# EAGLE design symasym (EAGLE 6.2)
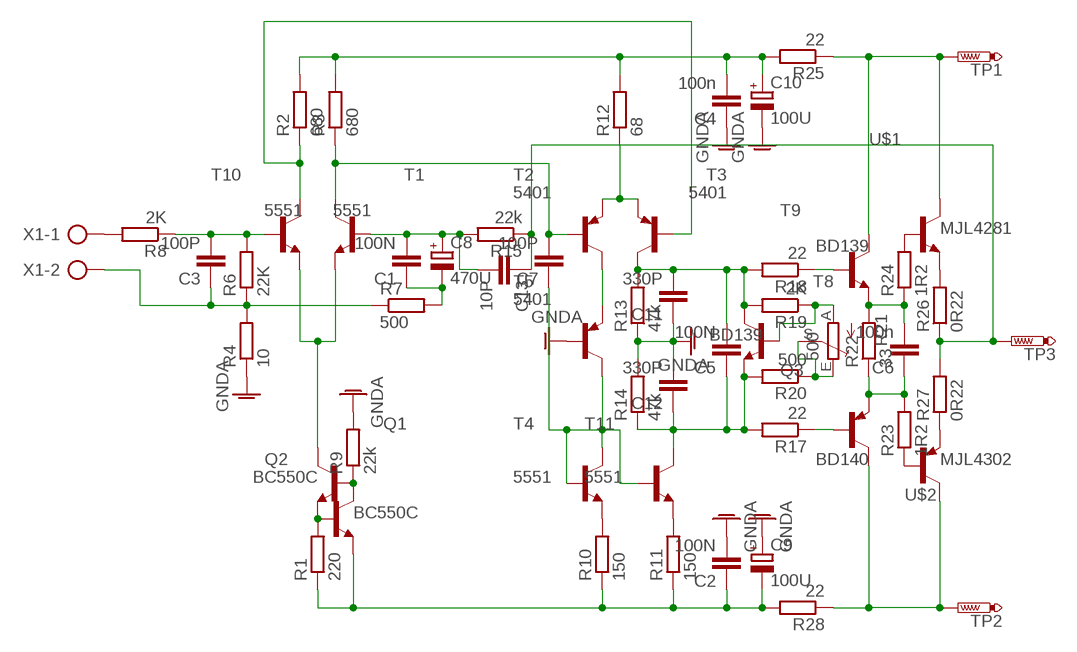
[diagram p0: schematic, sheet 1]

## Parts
C1  100N  C5/2.5  [C5B2.5]
C2  100N  C5/2.5  [C5B2.5]
C3  100P  C5/2.5  [C5B2.5]
C4  100n  C5/2.5  [C5B2.5]
C5  100N  C5/2.5  [C5B2.5]
C6  100n  C5/2.5  [C5B2.5]
C7  100P  C5/2.5  [C5B2.5]
C8  470U  CPOL-EUE5-13  [E5-13]
C9  100U  CPOL-EUE5-13  [E5-13]
C10  100U  CPOL-EUE5-13  [E5-13]
C11  330P  C5/2.5  [C5B2.5]
C12  330P  C5/2.5  [C5B2.5]
C13  10P  C5/2.5  [C5B2.5]
Q1  BC550C  [TO92-EBC]
Q2  BC550C  [TO92-EBC]
Q3  BD140  [TO126]
R1  220  R-EU_0207/12  [0207/12]
R2  680  R-EU_0207/12  [0207/12]
R3  680  R-EU_0207/12  [0207/12]
R4  10  R-EU_0207/12  [0207/12]
R6  22K  R-EU_0207/12  [0207/12]
R7  500  R-EU_0207/12  [0207/12]
R8  2K  R-EU_0207/12  [0207/12]
R9  22k  R-EU_0207/12  [0207/12]
R10  150  R-EU_0207/12  [0207/12]
R11  150  R-EU_0207/12  [0207/12]
R12  68  R-EU_0207/12  [0207/12]
R13  47k  R-EU_0207/12  [0207/12]
R14  47k  R-EU_0207/12  [0207/12]
R15  22k  R-EU_0207/10  [0207/10]
R17  22  R-EU_0207/12  [0207/12]
R18  22  R-EU_0207/10  [0207/10]
R19  2K  R-EU_0207/12  [0207/12]
R20  500  R-EU_0207/12  [0207/12]
R21  500  TRIM_EU-B64Y  [B64Y]
R22  33  R-EU_0411/15  [0411/15]
R23  1R2  R-EU_0411/15  [0411/15]
R24  1R2  R-EU_0411/15  [0411/15]
R25  22  R-EU_0411/15  [0411/15]
R26  0R22  R-EU_0922/22  [0922/22]
R27  0R22  R-EU_0922/22  [0922/22]
R28  22  R-EU_0411/15  [0411/15]
T1  5551  2N5551-NPN-TO92-EBC  [TO92-EBC]
T2  5401  2N5401-PNP-TO92-EBC  [TO92-EBC]
T3  5401  2N5401-PNP-TO92-EBC  [TO92-EBC]
T4  5551  2N5551-NPN-TO92-EBC  [TO92-EBC]
T5  5401  2N5401-PNP-TO92-EBC  [TO92-EBC]
T8  BD139  [TO126]
T9  BD139  [TO126]
T10  5551  2N5551-NPN-TO92-EBC  [TO92-EBC]
T11  5551  2N5551-NPN-TO92-EBC  [TO92-EBC]
TP1  PTR1PAD1-17Y  [P1-17Y]
TP2  PTR1PAD1-17Y  [P1-17Y]
TP3  PTR1PAD1-17Y  [P1-17Y]
U$1  MJL4281  [TO-264]
U$2  MJL4302  [TO-264]
X1  AK500/2  [AK500/2]

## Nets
GNDA: C2.2 C4.1 C9.+ C10.- C11.1 C12.2 R4.1 R9.2 R13.1 R14.2 T5.B
N$1: Q1.E Q2.B R1.2
N$2: Q1.B Q2.C R9.1
N$3: R2.1 T3.B T10.C
N$4: C3.1 R4.2 R6.1 R7.1 X1.2
N$5: C7.2 R3.1 T1.C T2.B
N$6: R10.2 T4.E
N$7: Q1.C T1.E T10.E
N$8: C4.2 C10.+ R2.2 R3.2 R12.2 R25.2
N$9: C3.2 R6.2 R8.1 T10.B
N$10: C7.1 T4.B T4.C T5.C T11.B
N$11: R11.2 T11.E
N$13: T2.C T5.E
N$14: R12.1 T2.E T3.E
N$15: C2.1 C9.- Q2.E R1.1 R10.1 R11.1 R28.2
N$16: C1.1 C8.- R7.2
N$17: C1.2 C8.+ C13.2 R15.2 T1.B
N$18: C5.1 C12.1 R14.1 R17.2 R20.2 T8.1(E) T11.C
N$19: C13.1 R15.1 R26.1 R27.2 TP3.TP
N$20: C5.2 C11.2 R13.2 R18.2 R19.2 T3.C T8.2(C)
N$21: R25.1 T9.2(C) TP1.TP U$1.C
N$23: R8.2 X1.1
N$24: Q3.2(C) R28.1 TP2.TP U$2.C
N$26: R19.1 R21.A T8.3(B)
N$27: R20.1 R21.E R21.S
N$28: R18.1 T9.3(B)
N$29: Q3.3(B) R17.1
N$30: C6.1 Q3.1(E) R22.1 R23.2
N$31: C6.2 R22.2 R24.1 T9.1(E)
N$32: R24.2 U$1.B
N$33: R23.1 U$2.B
N$34: R26.2 U$1.E
N$36: R27.1 U$2.E

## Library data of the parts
C1-C7 C11-C13 = capacitor-wima:C: CAPACITOR
C8-C10 = rcl:CPOL-EU: POLARIZED CAPACITOR, European symbol
Q1 Q2 = transistor-npn:BC550*: NPN Transistor
Q3 = transistor-pnp:BD140: PNP Transistor
R1-R4 R6-R15 R17-R20 R22-R28 = resistor:R-EU_: RESISTOR, European symbol
R21 = pot:TRIM_EU-: POTENTIOMETER
T1 T4 T10 T11 = transistor-neu-to92:*-NPN-: NPN Transistror
T2 T3 T5 = transistor-neu-to92:*-PNP-: PNP Transistror
T8 T9 = transistor:BD139: NPN TRANSISTOR
TP1-TP3 = testpad:PTR1: TEST PIN
U$1 = Rudi_TO264:MJL4281: MJL4281 NPN BCE TO-264
U$2 = Rudi_TO264:MJL4302: MJL4302 PNP BCE TO-264
X1 = con-ptr500:AK500/2: CONNECTOR; OC_FARNELL: unknown; OC_NEWARK: unknown

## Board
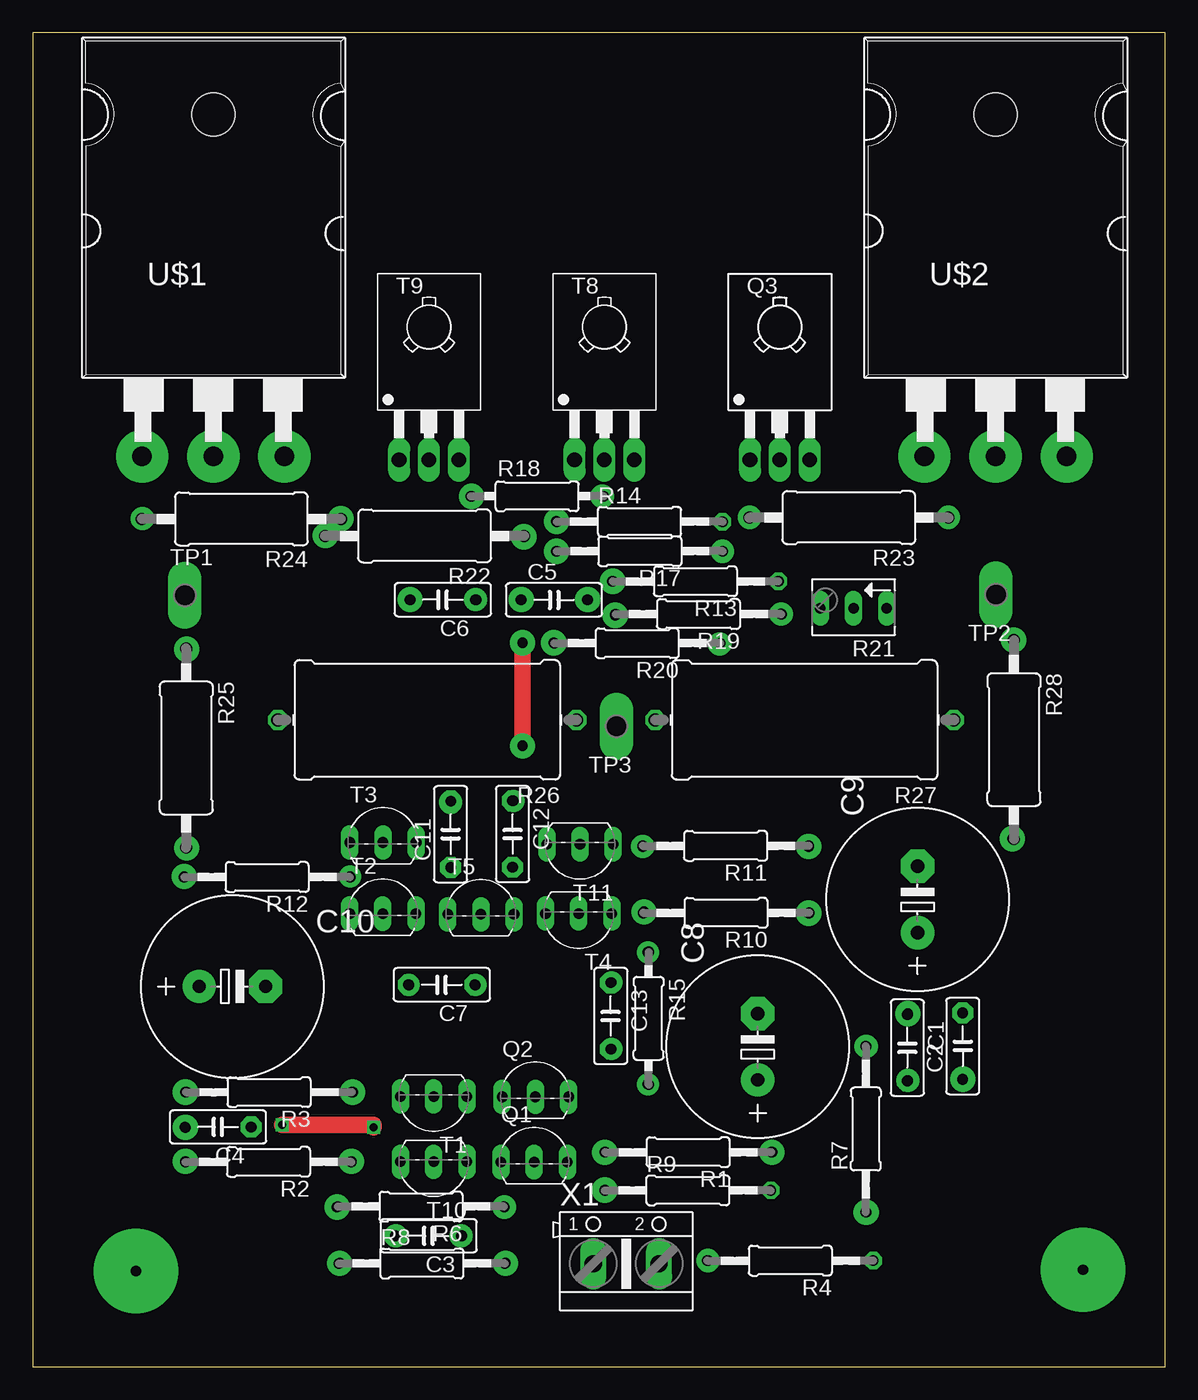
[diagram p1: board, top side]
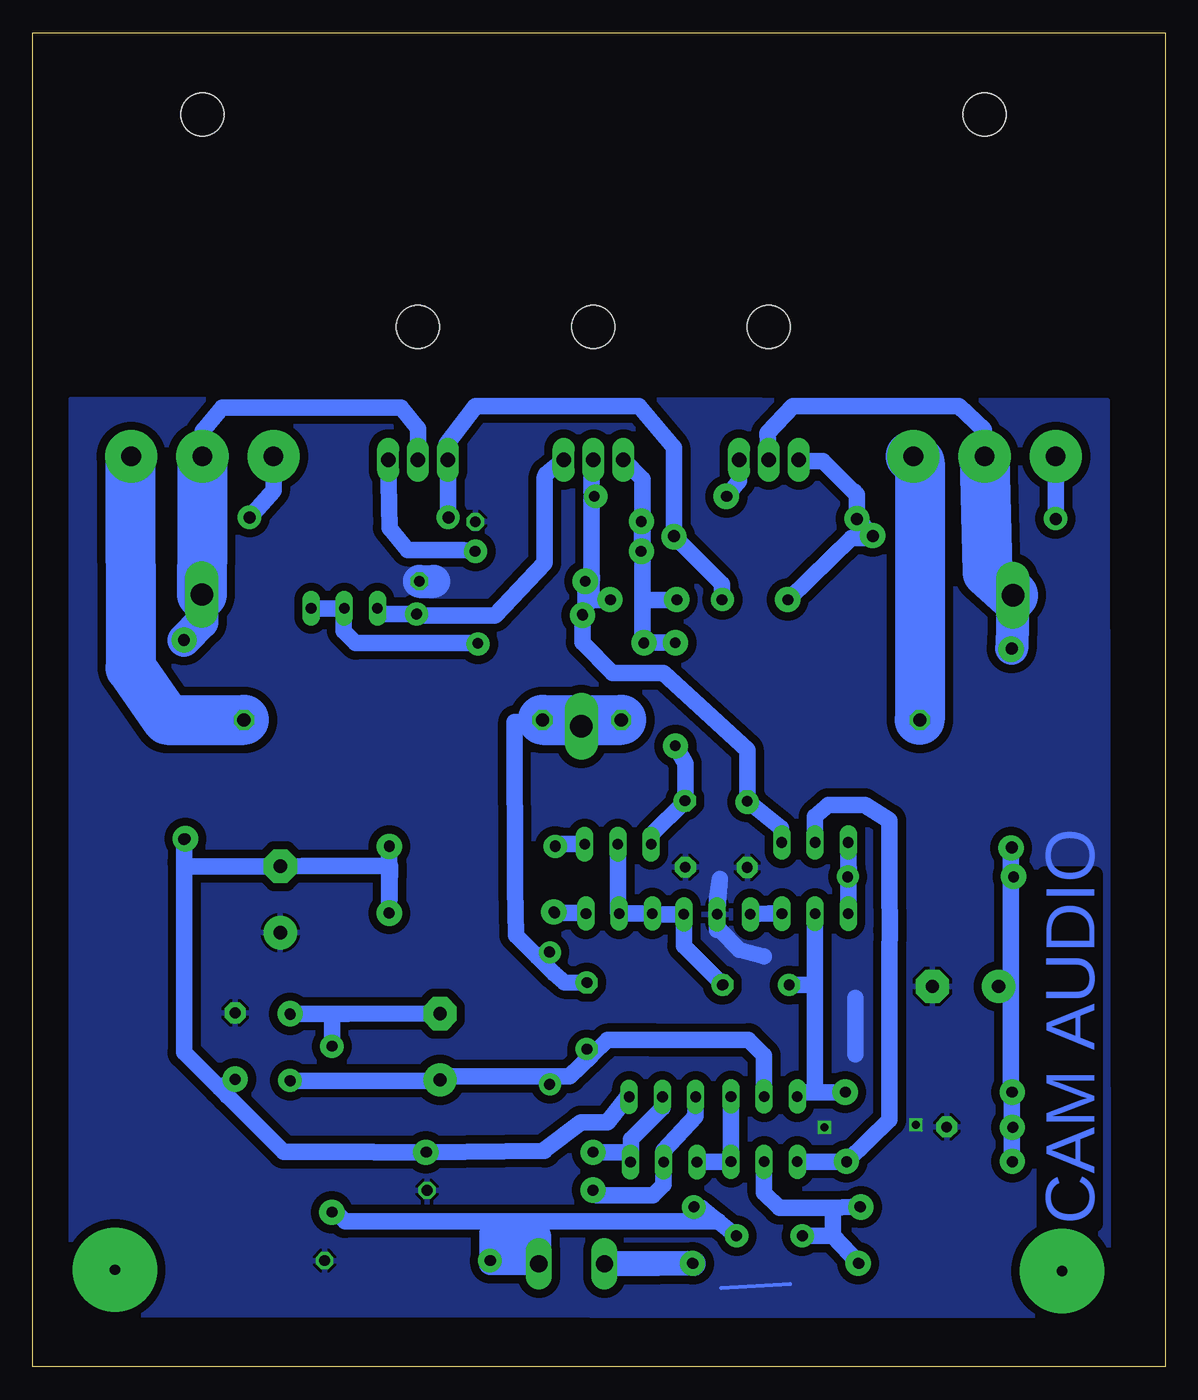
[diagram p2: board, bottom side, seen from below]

Size 86.7 x 102.13 mm. Coordinates in mm from the lower left corner, seen from the top.
Outline: 0,0 86.7,0 86.7,102.13 0,102.13 0,0
Copper layers (1*16): Top 0.035mm / dielectric 1.5mm / Bottom 0.035mm
Design rules: minimum track width 10mil, minimum drill 24mil, track to track 25mil, track to pad 25mil, pad to pad 25mil, via to via 25mil, smd to smd 25mil, copper to edge 40mil, drill to drill 8mil, minimum pad ring 10mil, minimum via ring 8mil, stop-mask expansion 4mil, vias tented up to drill 0mil, thermal gap 10mil

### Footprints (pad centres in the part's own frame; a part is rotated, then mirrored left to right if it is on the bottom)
C5B2.5 = drill 0.813 pad 1.6 octagon: 1 -2.54,0; 2 2.54,0
E5-13 = drill 1.016 pad 2.54: + -2.54,0 | drill 1.016 pad 2.54 octagon: - 2.54,0
TO92-EBC = drill 0.813 long: B 0,-1.27; C -2.54,-1.27; E 2.54,-1.27
TO126 = drill 1.118 long: 1 -2.286,-5.08; 2 0,-5.08; 3 2.286,-5.08 | hole 3.302: 0,5.08
0207/12 = drill 0.813 octagon: 1 -6.35,0; 2 6.35,0
0207/10 = drill 0.813 octagon: 1 -5.08,0; 2 5.08,0
B64Y = drill 0.813 long: A 2.54,0; E -2.54,0; S 0,0
0411/15 = drill 0.914 octagon: 1 -7.62,0; 2 7.62,0
0922/22 = drill 1.016 octagon: 1 -11.43,0; 2 11.43,0
TO92-EBC' = drill 0.813 long: B 0,-1.27; C 2.54,-1.27; E -2.54,-1.27
P1-17Y = drill 1.702 pad 2.121 long: TP 0,0
TO-264 = drill 1.5 pad 4: B -5.45,-6.096; E 5.45,-6.096 | drill 1.499 pad 4: C 0,-6.096 | hole 3.3: 0,20.09
AK500/2 = drill 1.321 long: 1 -2.515,0; 2 2.515,0

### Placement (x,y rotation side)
C1  66.96,24.43 270 top
C2  71.2,24.55 90 top
C3  30.31,10.03 180 top
C4  14.19,18.36 180 top
C5  39.91,58.71 0 top
C6  31.4,58.72 180 top
C7  31.32,29.25 180 top
C8  55.51,24.5 90 top
C9  67.74,35.78 90 top
C10  15.29,29.12 0 top
C11  32,40.77 90 top
C12  36.74,40.79 270 top
C13  44.25,26.86 270 top
Q1  38.39,16.94 0 top
Q2  38.49,21.94 0 top
Q3  57.2,74.52 0 top
R1  50.18,16.43 180 top
R2  18.05,15.69 180 top
R3  18.1,21.03 180 top
R4  58,8.13 180 top
R6  29.72,12.27 180 top
R7  63.78,18.2 90 top
R8  29.8,7.91 0 top
R9  50.16,13.51 0 top
R10  53.08,34.75 180 top
R11  53.05,39.88 180 top
R12  17.95,37.49 180 top
R13  50.74,60.13 180 top
R14  46.46,64.69 0 top
R15  47.15,26.68 270 top
R17  46.48,62.43 180 top
R18  38.62,66.64 0 top
R19  50.97,57.62 180 top
R20  46.28,55.39 180 top
R21  62.84,58.06 180 top
R22  30,63.6 180 top
R23  62.48,65 180 top
R24  15.98,64.9 180 top
R25  11.75,47.37 270 top
R26  30.21,49.52 180 top
R27  59.09,49.52 180 top
R28  75.12,48.01 270 top
T1  5551  [TO92-EBC']  30.7,19.43 180 top
T2  5401  [TO92-EBC']  26.8,35.96 0 top
T3  5401  [TO92-EBC']  26.81,41.41 0 top
T4  5551  [TO92-EBC']  41.8,33.43 180 top
T5  5401  [TO92-EBC']  34.31,35.91 0 top
T8  43.77,74.52 0 top
T9  30.34,74.52 0 top
T10  5551  [TO92-EBC']  30.7,14.43 180 top
T11  5551  [TO92-EBC']  41.9,38.73 180 top
TP1  11.65,59.07 0 top
TP2  73.75,59.12 180 top
TP3  44.7,49.03 180 top
U$1  13.83,75.79 0 top
U$2  73.71,75.79 0 top
X1  45.44,7.89 0 top

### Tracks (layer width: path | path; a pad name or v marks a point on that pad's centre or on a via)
GNDA  (via drill 0.6)
  Top 1.27: v19.1,18.53 26.1,18.53 v26.1,18.33
  Bottom 0.305: 28.7,6.33 34,6.03
  Bottom 1.27: 34.1,37.33 34.3,35.83 | 34.1,37.33 34.2,36.33 34.3,35.83 | 34.3,35.83 34.3,33.43 34.1,33.43 32.6,31.93 30.7,31.43 | 34.1,37.33 T5.B | 23.7,28.23 23.7,23.93
  Bottom 2.54: R13.1 56,60.13
  pour Bottom: 4.44,73.98 83.73,74.08 83.73,4 4.34,3.9
N$1
  Bottom 1.27: R1.2 40.89,16.43 Q1.E 40.9,15.7 40.9,17.43 38.49,19.84 Q2.B
N$2
  Bottom 1.27: Q2.C 35.95,19.18 38.39,16.54 Q1.B | Q1.B 38.41,15.47 | Q1.B 38.41,15.45 38.41,13.92 39.2,13.13 43.53,13.13 R9.1
N$3
  Bottom 1.27: T3.B 26.8,42.13 25.8,43.03 23,43.03 21.1,41.83 21.1,36.65 21.09,33.44 21.1,31.73 21.1,18.89 R2.1 27.8,15.69 27.81,15.7 T10.C
N$4
  Bottom 1.016: 48.9,10.43 48.9,11.13
  Bottom 1.27: C3.1 35.49,12.17 R6.1 34.21,11.13 48.9,11.13 62.8,11.13 63.52,11.85 R7.1
  Bottom 1.778: X1.2 51.65,7.89 R4.2 51.6,8.13 51.6,10.43 50.6,10.43 50.6,9.13 50,9.13 50,10.13 47.9,10.13 47.9,8.03 48.9,8.03 48.9,10.43
N$5  (via drill 0.8 pad 1.93)
  Bottom 1.27: R3.1 v24.5,21.03 26.7,21.03 | 26.7,21.03 28.16,21.03 T1.C | T2.B 26.8,28.73 | 26.8,28.73 26.8,21.13 26.7,21.03 | 26.8,28.73 26.82,29.25 C7.2
N$6
  Bottom 1.27: R10.2 44.6,34.73 44.4,34.76 T4.E
N$7
  Bottom 1.27: 33.25,21.07 T1.E T10.E 35.82,15.7 Q1.C
N$8
  Bottom 1.27: 11.75,18.36 R3.2 11.8,21.08 11.8,29.73 | 11.75,18.36 11.75,15.74 R2.2 | 11.8,29.73 11.8,37.33 | 11.8,37.33 11.8,39.5 R25.2 | C10.+ 11.81,29.12 11.8,29.73 | R12.2 11.76,37.39 11.8,37.33 | C4.2 11.75,18.36
N$9
  Bottom 1.27: 25.45,12.17 R6.2 25.36,12.16 | 25.45,12.17 25.45,10.03 | 25.45,10.03 R8.1 | 25.45,12.17 29.54,12.17 30.7,13.33 T10.B | C3.2 25.45,10.03
N$10
  Bottom 1.27: 36.8,34.69 T5.C | T5.C 39.19,34.63 T4.C T4.B 41.9,34.8 T11.B | T5.C 36.85,32.24 C7.1
N$11
  Bottom 1.27: R11.2 46.65,39.88 46.3,40.03 44.4,40.04 T11.E
N$12  (via drill 0.8 pad 1.78)
  other vias: 36.1,12.23
N$13
  Bottom 1.27: T2.C 30.32,34.69 T5.E
N$14
  Bottom 1.27: T3.E 24.27,38.13 | 24.27,38.13 T2.E | R12.1 24.21,38.19 24.27,38.13
N$15
  Bottom 1.27: R1.1 60.53,16.43 | Q2.E 41.16,20.67 42.7,18.73 44.73,18.73 47.5,16.63 47.5,16.53 R1.1 | R11.1 59.43,39.85 R10.1 59.33,38.33 66.05,38.33 C9.- 74.81,38.32 75.12,38.63 | R1.1 60.65,16.45 67.5,16.45 71.78,20.73 | 71.8,20.73 71.78,20.73 | R28.2 75.12,38.63 | 75.12,38.63 75.12,24.07 72.39,21.34 | 72.39,21.34 71.78,20.73 | C2.1 72.39,21.34
N$16
  Bottom 0.813: 63.78,26.94 62.6,27.02
  Bottom 1.27: C8.- 62.6,27.02 66.87,27.02 C1.1 | R7.2 63.78,26.94
N$17
  Bottom 0.406: R15.2 45.6,22.2 45.6,22.23 | C13.2 43.93,24.32 43.93,23.84
  Bottom 1.27: T1.B 30.7,23.83 31.9,25.03 39.2,25.03 39.29,25.02 42.71,25.02 43.93,23.84 45.6,22.23 55.66,22.23 C8.+ 55.97,21.9 C1.2
N$18  (via drill 0.8 pad 1.93)
  Top 1.27: v37.5,55.43 v37.5,47.53
  Bottom 1.27: 40,55.32 40,58.63 | 40,58.63 40,61.73 | 40,61.73 40,62.03 | 40,62.03 40,67.96 T8.1 | R14.1 40.01,62.04 arc-90 40,62.03 | R17.2 40.03,61.7 arc90 40,61.73 | 37.25,58.59 C5.1 39.92,58.71 40,58.63 | 40,55.32 40,55.23 39.9,55.43 v37.5,55.43 | 40,55.32 R20.2 | v37.5,47.53 36.74,46.17 C12.1 39.36,40.71 T11.C
N$19
  Bottom 1.27: R26.1 49.8,49.38 49.78,36.63 49.7,33.03 48.1,31.43 | C13.1 45.98,29.43 46.8,30.13 48.1,31.43 | TP3.TP 46.75,49.43 R27.2 | R15.1 48.1,31.43
  Bottom 3.81: R27.2 R26.1
N$20  (via drill 0.6 pad 1.78)
  Bottom 1.27: 43.9,60.13 43.9,58.63 43.82,58.71 C5.2 | 43.9,60.13 43.9,60.53 | T8.2 43.9,69.31 43.9,66.97 | 43.9,66.97 v43.6,66.63 43.9,66.63 43.9,60.53 | 43.87,60.25 43.87,60.5 43.9,60.53 | 43.9,60.13 R13.2 44.39,58.15 R19.2 44.62,55.45 42.3,53.13 38.4,53.13 32,47.23 C11.2 29.41,41.24 T3.C | 43.9,66.97 R18.2
N$21
  Bottom 1.27: T9.2 30.44,71.49 28.5,73.53 15.8,73.53 13.9,71.73 13.9,69.76 U$1.C | TP1.TP 11.65,58.97
  Bottom 2.54: 11.65,58.97 R25.1
  Bottom 3.81: U$1.C 13.6,60.83 TP1.TP
N$22  (via drill 0.8 pad 1.78)
  other vias: 27.8,10.03
N$23
  Bottom 1.93: R8.2 38.87,7.89 X1.1
N$24  (via drill 0.8 pad 1.93)
  Bottom 1.27: 74.9,63.33 73.6,64.63 v73.8,59.13 74.9,68.5 U$2.C 73.7,69.7 73.7,71.63 72.2,73.43 58.5,73.43 57.2,71.83 Q3.2
  Bottom 2.54: TP2.TP 73.75,57 R28.1
  Bottom 3.81: U$2.C 73.71,63.74 TP2.TP
N$25  (via drill 0.8 pad 1.78)
  other vias: 33.9,58.73
N$26
  Bottom 1.27: T8.3 47.39,68.34 47.5,68.03 47.5,61.53 51.3,57.53 57.33,57.53 R19.1 60.16,57.62 R21.A
N$27
  Bottom 1.27: R21.E R21.S 62.9,57.9 62.9,56.33 61.96,55.39 R20.1
N$28
  Bottom 1.27: T9.3 32.63,67.8 R18.1
N$29
  Bottom 1.27: Q3.3 59.39,64.22 58,62.53 53.7,62.53 52.93,62.4 52.9,62.43 R17.1
N$30
  Bottom 1.27: R23.2 54.91,65.55 Q3.1 55,69.53 55,70.63 52.8,73.53 40.3,73.53 37.62,70.35 R22.1 33.94,59.92 C6.1
N$31
  Bottom 1.27: T9.1 27.91,69.44 27.8,69.33 26.2,69.33 23.7,66.83 23.73,66.89 | 23.73,66.89 23.8,67 | R24.1 23.5,64.8 22.5,63.46 24.02,63.46 C6.2 | R24.1 23.6,66.75 23.73,66.89 | R22.2 23.28,64.6 R24.1
N$32
  Bottom 1.27: U$1.B 8.38,64.92 R24.2
N$33
  Bottom 1.27: U$2.B 68.26,67.06 R23.1
N$34
  Bottom 1.27: R26.2 18.79,51.52 18.8,49.53
  Bottom 3.81: U$1.E 19.48,69.71 18.8,69.23 18.8,49.53
N$35  (via drill 0.8 pad 1.68)
  other vias: 36.8,43.33
N$36
  Bottom 3.81: U$2.E 79.22,69.43 79.2,53.53 76.4,49.52 R27.1
N$37  (via drill 0.8 pad 1.68)
  other vias: 24.3,37.53
N$39  (via drill 0.8 pad 1.93)
  other vias: 8.4,69.73
N$40  (via drill 0.8 pad 1.93)
  other vias: 13.8,69.73
N$41  (via drill 0.8 pad 1.68)
  other vias: 47.1,31.73
N$42  (via drill 0.8 pad 1.68)
  other vias: 44.3,24.33
N$43  (via drill 0.8 pad 1.68)
  other vias: 44.3,29.43
N$44  (via drill 0.8 pad 1.68)
  other vias: 47.1,21.63
N$45  (via drill 0.8 pad 1.68)
  other vias: 33.9,29.23
N$46  (via drill 0.8 pad 1.68)
  other vias: 28.8,29.23
N$47  (via drill 0.8 pad 1.78)
  other vias: 57.3,57.63
N$48  (via drill 0.8 pad 1.93)
  other vias: 36.2,7.93
N$49  (via drill 0.8 pad 1.93)
  other vias: 23.5,7.93
N$50  (via drill 0.8 pad 1.78)
  other vias: 32.8,10.03
N$51  (via drill 0.8 pad 1.93)
  other vias: 56.6,16.43
N$52  (via drill 0.8 pad 1.78)
  other vias: 63.8,24.53
N$53  (via drill 0.8 pad 1.93)
  other vias: 23.3,12.23
N$54  (via drill 0.8 pad 1.93)
  other vias: 24.4,15.73
N$55  (via drill 0.8 pad 1.93)
  other vias: 11.7,21.03
N$56  (via drill 0.8 pad 1.93)
  other vias: 11.7,15.73
N$57  (via drill 0.8 pad 1.93)
  other vias: 11.7,18.33
N$58  (via drill 0.8 pad 1.78)
  other vias: 67,21.93
N$59  (via drill 0.8 pad 1.78)
  other vias: 51.7,8.13
N$62  (via drill 0.8 pad 1.93)
  other vias: 43.8,13.53
N$63  (via drill 0.8 pad 1.93)
  other vias: 63.8,11.83
N$64  (via drill 0.8 pad 1.93)
  other vias: 67,27.03
N$67  (via drill 0.6 pad 1.78)
  other vias: 44.7,49.03
N$68  (via drill 0.8 pad 1.93)
  other vias: 59.4,39.83
N$70  (via drill 0.8 pad 1.93)
  other vias: 37.4,58.73
N$71  (via drill 0.8 pad 1.93)
  other vias: 46.8,34.83
N$72  (via drill 0.6 pad 1.78)
  other vias: 70.1,65.03
N$73  (via drill 0.8 pad 1.93)
  other vias: 42.5,58.73
N$74  (via drill 0.8 pad 1.93)
  other vias: 40.1,62.43
N$75  (via drill 0.8 pad 1.93)
  other vias: 23.6,64.93
N$76  (via drill 0.8 pad 1.93)
  other vias: 11.8,54.93
N$77  (via drill 0.8 pad 1.93)
  other vias: 11.6,59.03
N$78  (via drill 0.8 pad 1.93)
  other vias: 33.6,66.63
N$79  (via drill 0.8 pad 1.93)
  other vias: 28.9,58.73
N$80  (via drill 0.8 pad 1.93)
  other vias: 59.4,34.73
N$81  (via drill 0.8 pad 1.93)
  other vias: 22.4,63.63
N$82  (via drill 0.8 pad 1.93)
  other vias: 44.4,60.13
N$83  (via drill 0.8 pad 1.93)
  other vias: 44.6,57.53
N$84  (via drill 0.8 pad 1.93)
  other vias: 37.6,63.53
N$85  (via drill 0.8 pad 1.93)
  other vias: 39.9,55.43
N$87  (via drill 0.6 pad 1.78)
  other vias: 54.9,65.03
N$88  (via drill 0.8 pad 1.93)
  other vias: 43.8,16.43
N$90  (via drill 0.8 pad 1.93)
  other vias: 75.1,55.63
N$91  (via drill 0.8 pad 1.93)
  other vias: 75,40.43
N$92  (via drill 0.8 pad 1.93)
  other vias: 71.2,22.03
N$94  (via drill 0.8 pad 1.93)
  other vias: 11.8,39.73
N$95  (via drill 0.8 pad 1.93)
  other vias: 11.6,37.53
N$96  (via drill 0.8 pad 1.93)
  other vias: 19.3,69.63
N$97  (via drill 0.8 pad 1.93)
  other vias: 68.3,69.63
N$98  (via drill 0.8 pad 1.93)
  other vias: 73.7,69.63
N$99  (via drill 0.8 pad 1.93)
  other vias: 79.2,69.73
N$100  (via drill 0.8 pad 1.78)
  other vias: 46.7,39.83
N$101  (via drill 0.8 pad 1.93)
  other vias: 63.8,11.83
N$102  (via drill 0.8 pad 1.93)
  other vias: 40.1,64.73
N$103  (via drill 0.8 pad 6.45)
  other vias: 7.9,7.33
N$104  (via drill 0.8 pad 6.45)
  other vias: 80.4,7.43
N$107  (via drill 0.8 pad 1.78)
  other vias: 8.4,64.93
N$108  (via drill 0.6 pad 1.78)
  other vias: 52.8,62.43
N$109  (via drill 0.6 pad 1.78)
  other vias: 52.6,55.33
N$110  (via drill 0.6 pad 1.78)
  other vias: 32,43.23

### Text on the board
Bottom: CAM AUDIO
